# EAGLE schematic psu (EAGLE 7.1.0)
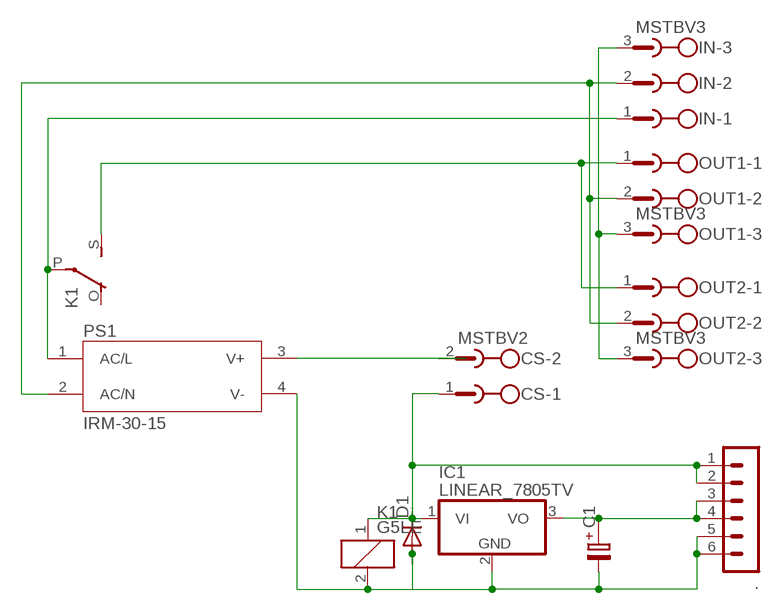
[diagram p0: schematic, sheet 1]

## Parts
.  MA06-1  [MA06-1]
C1  C-PR-2,0X5  [E2,0-5]
CS  MSTBV2  [MSTBV2]
D1  DIODE-D-2.5  [D-2.5]
IC1  LINEAR_7805TV  [LINEAR_TO220V]
IN  MSTBV3  [MSTBV3]
K1  G5LE  [G5LE]
OUT1  MSTBV3  [MSTBV3]
OUT2  MSTBV3  [MSTBV3]
PS1  IRM-30-15  [CONV_IRM-30-15]

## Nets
N$1: IN.1 K1.P(2:P) PS1.1(AC/L)
N$2: ..1 ..2 CS.1 D1.C IC1.1(VI) K1.1
N$3: K1.S(2:S) OUT1.1 OUT2.1
N$4: IN.2 OUT1.2 OUT2.2 PS1.2(AC/N)
N$5: IN.3 OUT1.3 OUT2.3
N$6: ..3 ..4 C1.+ IC1.3(VO)
N$7: CS.2 PS1.3(V+)
N$9: ..5 ..6 C1.- D1.A IC1.2(GND) K1.2 PS1.4(V-)
Unconnected: K1.O(2:O)

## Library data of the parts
. = con-lstb:MA06-1: PIN HEADER; OC_FARNELL: unknown; OC_NEWARK: unknown
C1 = cap-pan40:C-PR: POLARIZED ELECTROLYTIC/TANTALUM
CS = con-phoenix-508:MSTBV2: PHOENIX; MPN: MSTBV 2,5/2-GF-5.08; OC_FARNELL: 1792792; OC_NEWARK: 69R9845
D1 = diode:DIODE-: DIODE
IC1 = brakeflash-v2-rev_11:LINEAR_78*: Positive VOLTAGE REGULATOR Source: http://cache.national.com/ds/LM/LM78L05.pdf http://www.fairchildsemi.com/ds/LM/LM7805.pdf
IN OUT1 OUT2 = con-phoenix-508:MSTBV3: PHOENIX; MPN: MSTBV 2,5/3-GF-5.08; OC_FARNELL: 1792793; OC_NEWARK: 69R9846
K1 = relay:G5LE: RELAY 1 x switch, 10 A/120 V AC, 8 A/30 V DC, Omron; OC_FARNELL: unknown; OC_NEWARK: unknown
PS1 = IRM-30-15:IRM-30-15: AC-DC Single output Encapsulated power supply| PCB mount; Input 85-264VAC; Output 15VDC at 2A; Compact size Check prices; AVAILABILITY: Warning; DESCRIPTION: Enclosed AC DC Converters 1 Output 15V 2A 85 ~ 264 VAC Input; MF: MEAN WELL; MP: IRM-30-15; PACKAGE: DIP-4 Mean Well; PRICE: None; PURCHASE-URL: https://pricing.snapeda.com/search/part/IRM-30-15/?ref=eda

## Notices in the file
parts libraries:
cap-pan40: Copyright (C) 2004, Bob Starr
